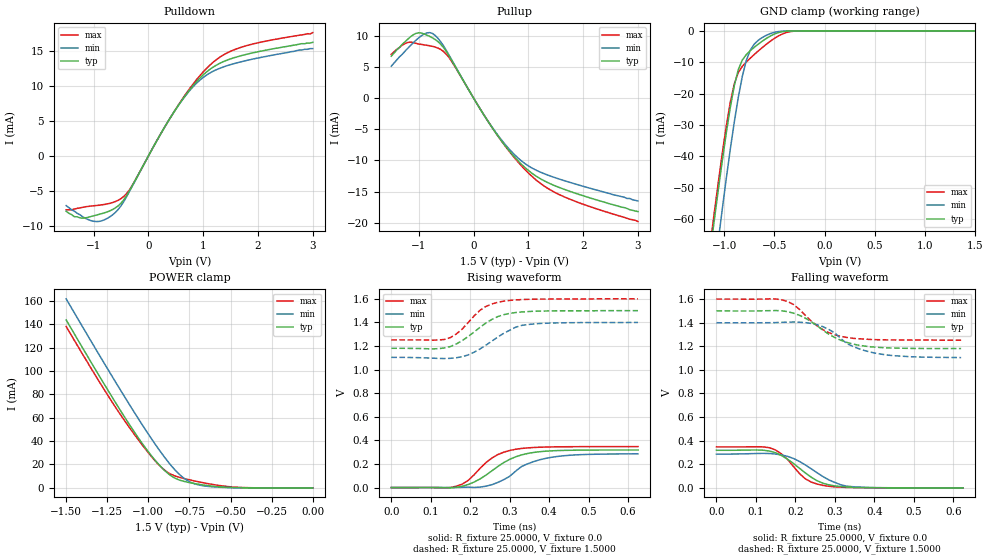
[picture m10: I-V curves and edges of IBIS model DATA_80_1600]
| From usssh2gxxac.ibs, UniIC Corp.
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|   Model DATA_80_1600
[Model]  DATA_80_1600
Model_type I/O
Polarity   Non-Inverting
Enable   Active-High
Vinl =   0.60000000V
Vinh =   0.90000000V
Vmeas =   0.750000000V
Rref =   25.00000000
Vref =   0.75000000V
C_comp   1.6160pF   1.5990pF   1.6430pF
[Temperature Range]   25.0000   95.0000   0.0
[Voltage Range]   1.5000V   1.4000V   1.6000V
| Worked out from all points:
|   slope of the pulldown table from 0 to 0.225 V, typ, clamps not added: 70.9 ohm
|   slope of the pullup table from 0 to 0.225 V, typ, clamps not added: 70 ohm
|   GND clamp passes 1 mA (typ) near -0.50 V on its own axis
|   POWER clamp passes 1 mA (typ) near -0.58 V on its own axis
|   rising waveform, R_fixture 25.0000, V_fixture 0.0: 20-80 % time 91.4ps typ, 90.7ps min, 71.4ps max; typ from 0 V to 0.318 V
|   rising waveform, R_fixture 25.0000, V_fixture 1.5000: 20-80 % time 82.5ps typ, 85.9ps min, 65.7ps max; typ from 1.18 V to 1.5 V
|   falling waveform, R_fixture 25.0000, V_fixture 0.0: 20-80 % time 79.1ps typ, 84.6ps min, 61.1ps max; typ from 0.318 V to 0 V
|   falling waveform, R_fixture 25.0000, V_fixture 1.5000: 20-80 % time 93.8ps typ, 90.3ps min, 77ps max; typ from 1.5 V to 1.18 V
[Pulldown]
|Voltage   I(typ)   I(min)   I(max)
-1.5V     -7.9mA     -7.1mA     -7.7mA
-1.25V    -8.86mA    -8.4mA     -7.43mA
-1V       -8.57mA    -9.35mA    -7.13mA
-800mV    -8.135mA   -9.13mA    -6.94mA
-600mV    -7.422mA   -8.068mA   -6.512mA
-350mV    -5.045mA   -5.146mA   -4.893mA
200mV     2.832mA    2.856mA    2.829mA
550mV     7.292mA    7.282mA    7.356mA
850mV     10.41mA    10.22mA    10.67mA
1.15V     12.59mA    12.03mA    13.23mA
1.7V      14.4mA     13.53mA    15.61mA
3V        16.3mA     15.4mA     17.7mA
[Pullup]
|Voltage   I(typ)   I(min)   I(max)
-1.5V     6.7mA      5.1mA      7mA
-1.25V    9mA        7.5mA      8.72mA
-1.05V    10.35mA    9.26mA     8.76mA
-900mV    10.25mA    10.25mA    8.51mA
-750mV    9.639mA    10.35mA    8.28mA
-600mV    8.621mA    9.028mA    7.779mA
-450mV    6.804mA    6.923mA    6.517mA
350mV     -4.882mA   -4.81mA    -4.873mA
900mV     -10.83mA   -10.26mA   -11.12mA
1.2V      -12.84mA   -11.81mA   -13.54mA
1.55V     -14.29mA   -12.95mA   -15.42mA
3V        -18.2mA    -16.5mA    -19.8mA
[GND_clamp]
|Voltage   I(typ)   I(min)   I(max)
-1.5V     -169mA     -189.1mA   -163.8mA
-1.14V    -70.71mA   -88.3mA    -68.32mA
-1.1V     -60.74mA   -77.66mA   -58.33mA
-1.06V    -51.03mA   -67.22mA   -48.61mA
-1.02V    -41.65mA   -57.06mA   -39.27mA
-940mV    -24.55mA   -37.9mA    -22.88mA
-860mV    -12.39mA   -21.26mA   -13.32mA
-780mV    -7.577mA   -9.433mA   -9.942mA
-740mV    -6.329mA   -6.125mA   -8.71mA
-620mV    -3.273mA   -2.113mA   -5.305mA
-300mV    -11.81uA   -4.878uA   -91.71uA
1.5V      4.577nA    23.6nA     33.33nA
[POWER_clamp]
|Voltage   I(typ)   I(min)   I(max)
-1.5V     143.7mA    161.7mA    138.1mA
-1.22V    77.56mA    95.29mA    73.32mA
-1.12V    55.19mA    72.34mA    52.54mA
-1.02V    34.59mA    50.23mA    33.56mA
-960mV    23.77mA    37.63mA    23.28mA
-900mV    14.66mA    25.9mA     15mA
-840mV    8.415mA    15.63mA    10.28mA
-780mV    5.408mA    7.848mA    7.861mA
-700mV    3.206mA    2.693mA    5.332mA
-600mV    1.29mA     794.5uA    2.681mA
-420mV    69.47uA    44.47uA    238.7uA
0V        4.577nA    6.249nA    39.08nA
[Ramp]
| variable   typ   min   max
dV/dt_r  0.1912/91.4560p   0.1717/0.1057n   0.2083/71.3681p
dV/dt_f  0.1914/93.7667p   0.1776/0.1053n   0.2088/77.0400p
R_load = 25.0000
[Rising Waveform]
R_fixture= 25.0000
V_fixture= 0.0
V_fixture_min= 0.0
V_fixture_max= 0.0
|time   V(typ)   V(min)   V(max)
0s        0V         0V         0V
165ps     2.02mV     524.9uV    11.92mV
195ps     25.97mV    3.571mV    60.83mV
255ps     142.2mV    24.51mV    250.4mV
300ps     239.2mV    95.42mV    314.5mV
315ps     260.6mV    138.9mV    324.6mV
330ps     276.7mV    178.3mV    331.6mV
360ps     297.5mV    219.5mV    339.6mV
420ps     313.4mV    263.4mV    345.4mV
625ps     318.5mV    286.1mV    347.2mV
[Rising Waveform]
R_fixture= 25.0000
V_fixture= 1.5000
V_fixture_min= 1.4000
V_fixture_max= 1.6000
|time   V(typ)   V(min)   V(max)
0s        1.181V     1.104V     1.252V
120ps     1.178V     1.095V     1.251V
150ps     1.196V     1.096V     1.272V
180ps     1.247V     1.11V      1.345V
225ps     1.359V     1.176V     1.504V
255ps     1.426V     1.242V     1.557V
285ps     1.466V     1.308V     1.581V
315ps     1.484V     1.359V     1.591V
360ps     1.495V     1.387V     1.597V
625ps     1.5V       1.4V       1.6V
[Falling Waveform]
R_fixture= 25.0000
V_fixture= 0.0
V_fixture_min= 0.0
V_fixture_max= 0.0
|time   V(typ)   V(min)   V(max)
0s        318.5mV    285.8mV    347.2mV
135ps     311.3mV    290.9mV    339.5mV
165ps     274mV      279mV      287mV
195ps     207.1mV    249.4mV    181.8mV
225ps     127.1mV    194.7mV    77.18mV
240ps     90.47mV    161.8mV    49.29mV
270ps     39.08mV    95.37mV    20.39mV
315ps     10.66mV    26.07mV    5.464mV
345ps     4.654mV    9.695mV    2.273mV
625ps     0V         0V         0V
[Falling Waveform]
R_fixture= 25.0000
V_fixture= 1.5000
V_fixture_min= 1.4000
V_fixture_max= 1.6000
|time   V(typ)   V(min)   V(max)
0s        1.5V       1.4V       1.6V
150ps     1.503V     1.401V     1.601V
180ps     1.494V     1.404V     1.58V
225ps     1.439V     1.401V     1.463V
270ps     1.336V     1.366V     1.34V
300ps     1.274V     1.313V     1.297V
330ps     1.233V     1.224V     1.275V
375ps     1.202V     1.164V     1.261V
435ps     1.186V     1.125V     1.254V
620ps     1.181V     1.104V     1.252V
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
